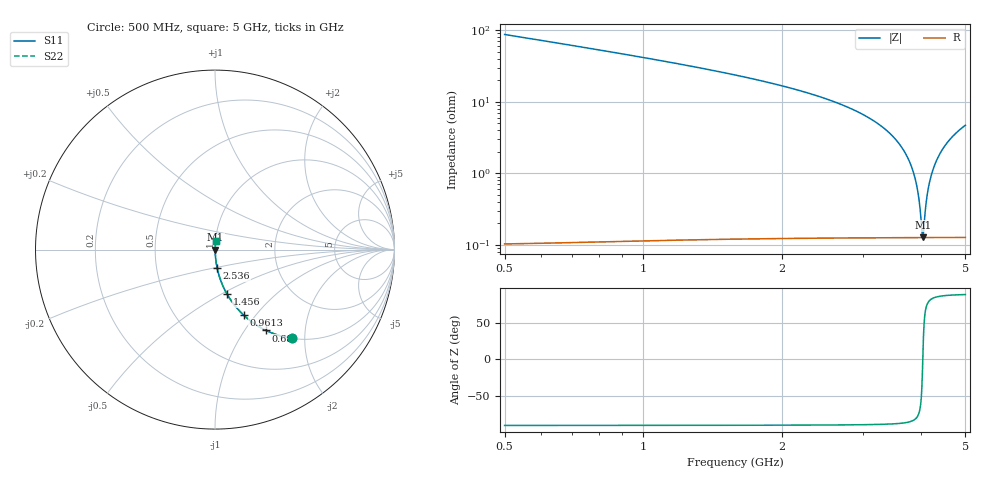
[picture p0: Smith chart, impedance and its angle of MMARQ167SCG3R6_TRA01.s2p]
! MMARQ167SCG3R6_TRA01  S-PARAMETER MODEL  ( General Type )
! Model Generated by TAIYO YUDEN Corporation (http://www.ty-top.com)
! Version 1.0
! TAIYO YUDEN Control No. 160201
! Copyright(c) 2016 TAIYO YUDEN CO.,LTD. All Rights Reserved.
! Product Description (link to TY-COMPAS)
! https://ds.yuden.co.jp/TYCOMPAS/or/detail?pn=MMARQ167SCG3R6BTRA01&u=M
! Products Name : Multilayer Ceramic Capacitors
! Characteristics :
!  Capacitance : 3.6 pF , Rated Voltage : 250V , TCC : CG / C0G
!  Case Size : 1.6 x 0.8 / 0.063 x 0.031 [mm/inch] , Thickness : 0.7 / 0.028 [mm/inch]
!  (Conditions: Temperature = 25 degC , DC Bias Current/Voltage = 0A / 0V)
! External Node Assignments :
!  1  o---| |---o  2
! GND o---------o GND
! Frequency Range : 500MHz  -  5000MHz  [ 401 STEP ]
# MHz S RI R 50
! Freq[MHz].  S11 Real  S11 Imag  S21 Real  S21 Imag  S12 Real  S12 Imag  S22 Real  S22 Imag
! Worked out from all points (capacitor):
!   401 points, 500 MHz to 5 GHz, reference 50 ohm
!   read as one part in series: C = 3.6 pF near 522.5 MHz
!   lowest |Z| = 127 mohm at 4.044 GHz (marker M1)
!   series resonance near 4.041 GHz, so ESL is about 430 pH
!   S11 on the Smith chart (normalised r, x): 500 MHz: 1.00, -1.74; 680 MHz: 1.00, -1.26; 961.2 MHz: 1.00, -0.87; 1.456 GHz: 1.00, -0.53; 2.536 GHz: 1.00, -0.21; 5 GHz: 1.00, +0.09
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500  0.4309 -0.4946  0.5691 0.4946  0.5691 0.4946  0.4309 -0.4946
680  0.2852 -0.4507  0.7148 0.4507  0.7148 0.4507  0.2852 -0.4507
961.25  0.1588 -0.3642  0.8412 0.3642  0.8412 0.3642  0.1588 -0.3642
1253.75  0.0929 -0.2884  0.9071 0.2884  0.9071 0.2884  0.0929 -0.2884
1456.25  0.0661 -0.2461  0.9339 0.2461  0.9339 0.2461  0.0661 -0.2461
2007.5  0.0278 -0.1609  0.9722 0.1609  0.9722 0.1609  0.0278 -0.1609
2536.25  0.0122 -0.1041  0.9878 0.1041  0.9878 0.1041  0.0122 -0.1041
2750  0.0086 -0.0854  0.9914 0.0854  0.9914 0.0854  0.0086 -0.0854
3188.75  0.00397 -0.052  0.996 0.052  0.996 0.052  0.00397 -0.052
3503.75  0.00223 -0.0312  0.9978 0.0312  0.9978 0.0312  0.00223 -0.0312
3717.5  0.00159 -0.0182  0.9984 0.0182  0.9984 0.0182  0.00159 -0.0182
3863.75  0.00136 -0.00977  0.9986 0.00977  0.9986 0.00977  0.00136 -0.00977
3942.5  0.00129 -0.00537  0.9987 0.00537  0.9987 0.00537  0.00129 -0.00537
3976.25  0.00128 -0.00351  0.9987 0.00351  0.9987 0.00351  0.00128 -0.00351
4021.25  0.00126 -0.00106  0.9987 0.00106  0.9987 0.00106  0.00126 -0.00106
4043.75  0.00126 0.000157  0.9987 -0.000157  0.9987 -0.000157  0.00126 0.000157
4055  0.00126 0.000763  0.9987 -0.000763  0.9987 -0.000763  0.00126 0.000763
4145  0.00129 0.00555  0.9987 -0.00555  0.9987 -0.00555  0.00129 0.00555
4257.5  0.00139 0.0114  0.9986 -0.0114  0.9986 -0.0114  0.00139 0.0114
4381.25  0.00158 0.0176  0.9984 -0.0176  0.9984 -0.0176  0.00158 0.0176
4538.75  0.00191 0.0254  0.9981 -0.0254  0.9981 -0.0254  0.00191 0.0254
5000  0.00346 0.0467  0.9965 -0.0467  0.9965 -0.0467  0.00346 0.0467
